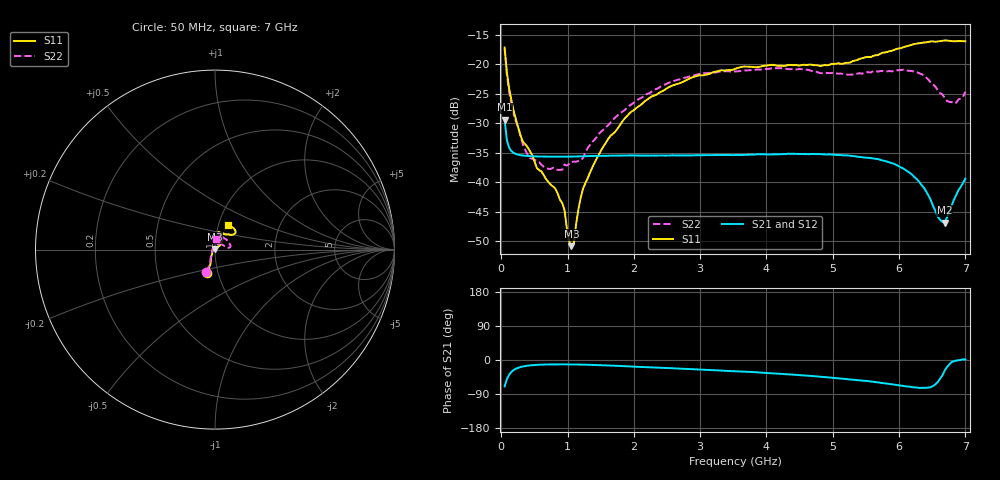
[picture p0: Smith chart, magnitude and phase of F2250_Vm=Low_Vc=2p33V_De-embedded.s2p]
! Integrated Device Technology
! Corporate Headquarters
! 6024 Silver Creek Valley Road
! San Jose, CA 95138  USA
! Phone:  1-408-284-8200
! Toll Free:  1-800-223-1366
! Webpage:  http://www.idt.com/
! Timing and RF Division
! 515 Groton Road, Suite 102
! Westford, MA 01886-6024
! Device:  F2250
! Description: Voltage Variable RF Attenuator
! Frequency:  50.0 -  6000.00 MHz
! Package:  3x3 mm Thin QFN Plastic Package: 16 pin
! Ports:  2 RF, 3 DC
!  Pin  1  = GND
!  Pin  2  = NC
!  Pin  3  = RF1  = Port 1
!  Pin  4  = NC
!  Pin  5  = GND
!  Pin  6  = GND
!  Pin  7  = GND
!  Pin  8  = GND
!  Pin  9  = NC
!  Pin 10  = RF2  = Port 2
!  Pin 11  = NC
!  Pin 12  = GND
!  Pin 13  = GND
!  Pin 14  = VCNTRL
!  Pin 15  = VDD
!  Pin 16  = VMODE
! Vcntrl:  2.330 Volts
! Vmode:  +0.000 Volts
! Vdd:  +3.30  Volts
! Current:  1.176 mA
! Data:  The device was measured on a the F2250 evaluation board which has
!  individual transmission lines to the RF pins.  Data was collected
!  using a calibrated network analyzer.  The evaluation board was
!  de-embedded using a TRL calibration technique.
!  The reference plane is the edge of the package pin.
! Misc:  SN 10
!  Action Tracker AT0258
! Date Measured:  2014-11-26
! Date:  2015-10-15  MJV
! Note:
!  Integrated Device Technology supplies this data as a sample of measured
!  data at the package pin for this product.  Your particular data for this
!  product may vary.
!  Data was taken at 25 degrees C.
!  Integrated Device Technology reserves the right to change this data at anytime.
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# GHz S dB R 50
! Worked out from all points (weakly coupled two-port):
!   201 points, 50 MHz to 7 GHz, reference 50 ohm
!   highest |S21| = -29.41 dB at 50 MHz (marker M1); lowest = -46.8 dB at 6.687 GHz (marker M2)
!   lowest |S11| = -50.8 dB at 1.058 GHz (marker M3), VSWR 1.01, Z = 49.8 + j0.24 ohm
!   |S11| at or under -10 dB: start of sweep to end of sweep
!   |S22| runs from -37.9 to -17.3 dB; largest |S21 - S12| = 6.1e-05
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0.05  -17.18 -108.6  -29.41 -69.7  -29.40 -69.7  -17.30 -110.9
0.08475  -21.45 -107.5  -32.90 -50.3  -32.90 -50.3  -21.79 -109.8
0.15425  -26.23 -116.6  -34.74 -31.1  -34.73 -31.1  -26.90 -121.8
0.29325  -32.20 -127.8  -35.41 -18.4  -35.41 -18.4  -32.27 -136.4
0.3975  -34.08 -141.9  -35.54 -15.0  -35.54 -15.0  -35.35 -159.6
0.5365  -37.57 -155.5  -35.61 -12.8  -35.61 -12.8  -36.41 178.3
0.91875  -43.50 158.1  -35.66 -11.5  -35.66 -11.5  -37.87 131.9
0.9535  -44.68 169.9  -35.66 -11.5  -35.66 -11.5  -36.97 129.7
1.023  -49.94 143.8  -35.65 -11.6  -35.65 -11.6  -36.87 114.0
1.05775  -50.80 123.3  -35.65 -11.6  -35.64 -11.6  -36.52 108.8
1.0925  -50.41 89.1  -35.63 -11.7  -35.63 -11.7  -36.50 104.1
1.162  -44.64 56.5  -35.62 -11.9  -35.61 -11.9  -36.38 93.3
1.2315  -41.13 44.5  -35.59 -12.1  -35.59 -12.1  -35.88 83.7
1.6485  -32.11 42.1  -35.50 -14.6  -35.50 -14.7  -29.88 63.4
2.37825  -24.87 47.4  -35.46 -20.3  -35.46 -20.3  -24.00 56.3
3.525  -20.80 72.5  -35.38 -29.6  -35.38 -29.6  -21.24 74.5
4.7065  -20.17 72.4  -35.19 -42.5  -35.19 -42.6  -21.20 72.1
5.85325  -17.82 40.5  -36.62 -63.3  -36.62 -63.4  -21.16 22.7
6.27025  -16.50 40.1  -39.47 -72.6  -39.48 -72.6  -21.38 9.3
6.68725  -15.99 48.8  -46.80 -28.2  -46.78 -27.8  -25.70 28.2
6.861  -16.13 55.1  -42.16 -1.5  -42.13 -1.6  -26.54 57.9
7  -16.12 63.2  -39.35 1.6  -39.30 1.6  -24.68 83.3
